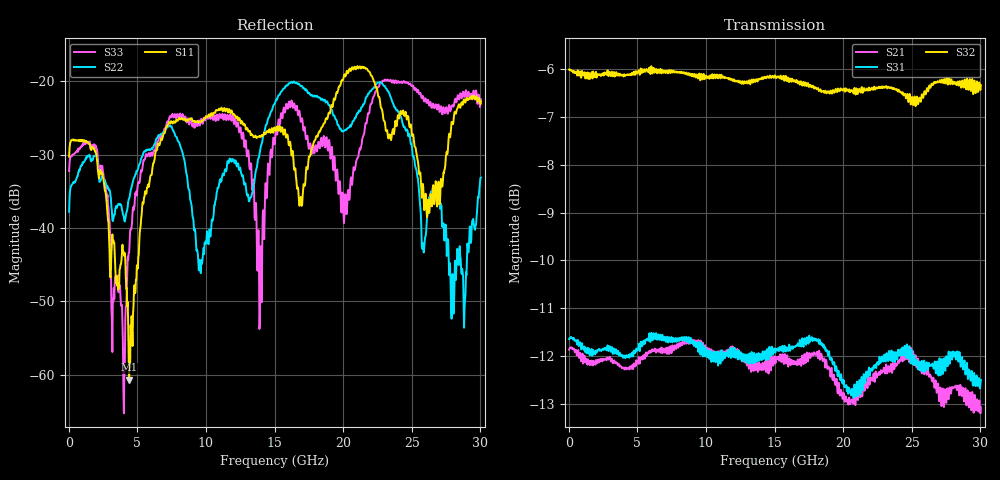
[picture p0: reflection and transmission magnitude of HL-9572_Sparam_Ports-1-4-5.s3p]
# GHZ S RI R 50.0
!; PortSelection: Port_123
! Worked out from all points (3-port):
!   858 points, 35 MHz to 30.03 GHz, reference 50 ohm
!   strongest paths, dB at 35 MHz, 7.525 GHz, 15.05 GHz, 22.54 GHz, 30.03 GHz:
!     S32: -6.0, -6.0, -6.2, -6.4, -6.3
!     S31: -11.7, -11.7, -11.9, -12.1, -12.5
!     S21: -11.9, -11.9, -12.2, -12.4, -13.1
!   lowest |S11| = -60.7 dB at 4.41 GHz (marker M1), VSWR 1.00, Z = 50.1 + j0.0225 ohm
!   |S11| at or under -10 dB: start of sweep to end of sweep
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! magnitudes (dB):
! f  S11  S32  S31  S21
! 35 MHz  -30.3  -6.0  -11.7  -11.9
! 4.41 GHz  -60.7  -6.1  -12.0  -12.3
! 7.21 GHz  -26.2  -6.0  -11.7  -11.9
! 9.59 GHz  -25.5  -6.2  -12.0  -11.7
! 13.96 GHz  -27.6  -6.2  -12.0  -12.2
! 15.05 GHz  -26.7  -6.2  -11.9  -12.2
! 20.16 GHz  -19.3  -6.4  -12.7  -12.9
! 22.93 GHz  -25.2  -6.4  -12.1  -12.3
! 27.96 GHz  -25.7  -6.3  -12.0  -12.7
! 30.03 GHz  -22.8  -6.3  -12.5  -13.1
